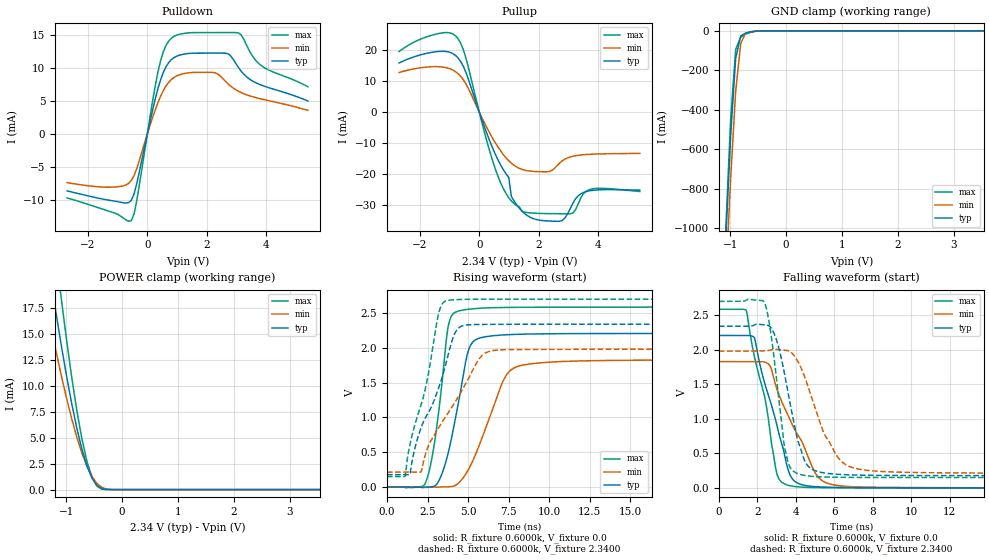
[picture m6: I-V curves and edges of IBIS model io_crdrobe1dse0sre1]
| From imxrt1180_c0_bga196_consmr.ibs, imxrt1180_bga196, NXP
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[Model]  io_crdrobe1dse0sre1
|   Model io_crdrobe1dse0sre1
| This model was characterised for following simulation conditions:
| External (pad) voltage:
|   - Typ: 2.34V,   - Min: 1.98V,   - Max: 2.7V
| Library cells for typ/min/max conditions are connected as defined below:
|  PAD_IO - External Pad
|  ipp_do - Core Input
|  ipp_obe - Output Buffer Enable
|  ASRCN3V3[3] - NC
|  ASRCN3V3[4] - NC
|  ASRCP3V3[4] - NC
|  REFAPBIAS3V3 - gnde
|  REFBAMPL3V3 - vdd1v8
|  REFCAMPH3V3 - vdd1v8
|  REFDNBIAS3V3 - vdd1v8
|  REFH3V3 - REFH3V3
|  REFL3V3 - REFL3V3
|  gnde - gnde
|  ipp_dse - gnde
|  ipp_ina235_3v - NC
|  ipp_ina40_3v - NC
|  ipp_ina_mux - NC
|  ipp_ind - NC
|  ipp_ind_1p8v - NC
|  ipp_ind_3v - NC
|  ipp_sre - vdd
|  vdd - vdd
|  vdd1v8 - vdd1v8
|  vdda - vdde3v3
|  vdde3v3 - vdde3v3
| All other pins connected to ground
Model_type I/O
Polarity   Non-Inverting
Enable   Active-High
Vinl =   0.7020V
Vinh =   1.6300V
Vmeas =  1.1700V
Cref =   15.0000pF
Rref =   0.6000k
Vref =   0.0V
C_comp   3.9951pF   3.8194pF   4.1033pF
|C_comp_pullup   0.5141pF   0.5881pF   0.4995pF
|C_comp_pulldown   2.0717pF   2.1609pF   1.8543pF
[Model Spec]
| variable   typ   min   max
Vinh   1.6300V   NA   NA
Vinl   0.7020V   NA   NA
Vref   0.0V   0.0V   0.0V
Cref   15.0000pF   15.0000pF   15.0000pF
Rref   0.6000k   0.6000k   0.6000k
[Receiver Thresholds]
Vcross_high  =   0.0V
Vcross_low  =   0.0V
Vdiff_ac  =   0.0V
Vdiff_dc  =   0.0V
Tdiffslew_ac  =   0.0S
[Temperature Range]   25.0000   0.1250k   -40.0000
[Voltage Range]   2.3400V   1.9800V   2.7000V
[Pullup Reference]   2.3400V   1.9800V   2.7000V
[Pulldown Reference]   0.0V   0.0V   0.0V
[POWER Clamp Reference]   2.3400V   1.9800V   2.7000V
[GND Clamp Reference]   0.0V   0.0V   0.0V
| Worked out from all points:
|   slope of the pulldown table from 0 to 0.351 V, typ, clamps not added: 51.9 ohm
|   slope of the pullup table from 0 to 0.351 V, typ, clamps not added: 37.8 ohm
|   GND clamp passes 1 mA (typ) near -0.49 V on its own axis
|   POWER clamp passes 1 mA (typ) near -0.53 V on its own axis
|   rising waveform, R_fixture 0.6000k, V_fixture 0.0: 20-80 % time 1.1ns typ, 1.77ns min, 787ps max; typ from 0 V to 2.21 V
|   rising waveform, R_fixture 0.6000k, V_fixture 2.3400: 20-80 % time 2ns typ, 2.66ns min, 1.49ns max; typ from 0.177 V to 2.34 V
|   falling waveform, R_fixture 0.6000k, V_fixture 0.0: 20-80 % time 1.29ns typ, 1.78ns min, 1.09ns max; typ from 2.21 V to 0 V
|   falling waveform, R_fixture 0.6000k, V_fixture 2.3400: 20-80 % time 975ps typ, 1.48ns min, 648ps max; typ from 2.34 V to 0.177 V
[Pulldown]
|Voltage   I(typ)   I(min)   I(max)
-2.7V     -8.67mA    -7.41mA    -9.74mA
-1.17V    -10.17mA   -8.095mA   -11.93mA
-540mV    -10.08mA   -7.082mA   -13.18mA
-360mV    -7.618mA   -5.325mA   -10.21mA
360mV     6.913mA    4.777mA    9.448mA
630mV     10.2mA     7.277mA    13.44mA
900mV     11.57mA    8.553mA    14.79mA
2.25V     12.24mA    9.288mA    15.36mA
2.7V      12.17mA    7.637mA    15.36mA
3.06V     10.09mA    6.461mA    15.32mA
3.78V     7.479mA    5.34mA     10.54mA
5.4V      4.985mA    3.556mA    7.138mA
[Pullup]
|Voltage   I(typ)   I(min)   I(max)
-2.7V     15.88mA    12.82mA    19.56mA
-1.44V    19.54mA    14.7mA     25.24mA
-720mV    17.58mA    12.48mA    23.82mA
-450mV    12.84mA    9.141mA    17.52mA
630mV     -15.42mA   -11.25mA   -20.73mA
990mV     -21.04mA   -15.7mA    -27.62mA
1.08V     -27.24mA   -16.49mA   -28.69mA
1.44V     -31.99mA   -18.49mA   -32.03mA
2.7V      -35.24mA   -16.46mA   -32.81mA
3.15V     -29.4mA    -14.24mA   -32.57mA
3.51V     -25.93mA   -13.74mA   -26.26mA
5.4V      -25.18mA   -13.3mA    -25.63mA
[GND_clamp]
|Voltage   I(typ)   I(min)   I(max)
-2.7V     -12.91A    -12.88A    -13.56A
-1.08V    -1.077A    -1.286A    -1.025A
-990mV    -533.6mA   -749.4mA   -449.1mA
-900mV    -139.2mA   -307mA     -94.25mA
-810mV    -25.49mA   -63.91mA   -32.87mA
-720mV    -11.78mA   -11.41mA   -16.65mA
-540mV    -1.684mA   -1.901mA   -2.149mA
-360mV    -36.04uA   -133.3uA   -15.05uA
5.4V      0A         0A         0A
[POWER_clamp]
|Voltage   I(typ)   I(min)   I(max)
-2.7V     73.96mA    57.58mA    95.4mA
-1.44V    26.15mA    20.18mA    34.67mA
-1.35V    22.86mA    17.7mA     30.34mA
-1.26V    19.66mA    15.3mA     26.09mA
-1.17V    16.56mA    12.98mA    21.97mA
-1.08V    13.59mA    10.78mA    17.99mA
-900mV    8.212mA    6.776mA    10.73mA
-720mV    3.9mA      3.518mA    4.888mA
-630mV    2.284mA    2.252mA    2.724mA
-540mV    1.103mA    1.268mA    1.195mA
-360mV    77.93uA    204.3uA    41.52uA
5.4V      0A         0A         0A
[Ramp]
| variable   typ   min   max
dV/dt_r  1.3244/1.0982n   1.0970/1.7718n   1.5519/0.7865n
dV/dt_f  1.2978/0.9748n   1.0605/1.4843n   1.5299/0.6476n
R_load = 0.6000k
[Rising Waveform]
R_fixture= 0.6000k
V_fixture= 0.0
V_fixture_min= 0.0
V_fixture_max= 0.0
|time   V(typ)   V(min)   V(max)
0s        133.2nV    3.451uV    44.06nV
2.399ns   -1.746mV   -5.701mV   74.77mV
2.994ns   21.55mV    -2.011mV   736mV
3.785ns   499.2mV    2.221mV    2.32V
4.667ns   1.562V     123.1mV    2.543V
5.021ns   1.966V     250.8mV    2.554V
5.443ns   2.114V     457.5mV    2.564V
7.306ns   2.187V     1.588V     2.58V
8.814ns   2.199V     1.769V     2.583V
60ns      2.207V     1.828V     2.587V
[Rising Waveform]
R_fixture= 0.6000k
V_fixture= 2.3400
V_fixture_min= 1.9800
V_fixture_max= 2.7000
|time   V(typ)   V(min)   V(max)
0s        177mV      212.5mV    150.2mV
1.117ns   176mV      212.4mV    151.9mV
1.418ns   183.8mV    211.9mV    614.9mV
2.104ns   853.1mV    216.7mV    1.183V
3.169ns   1.414V     847.7mV    2.479V
3.727ns   1.859V     1.049V     2.682V
4.48ns    2.299V     1.331V     2.695V
5.79ns    2.336V     1.874V     2.699V
6.922ns   2.338V     1.97V      2.7V
60ns      2.34V      1.98V      2.7V
[Falling Waveform]
R_fixture= 0.6000k
V_fixture= 0.0
V_fixture_min= 0.0
V_fixture_max= 0.0
|time   V(typ)   V(min)   V(max)
0s        2.207V     1.828V     2.586V
1.408ns   2.208V     1.828V     2.572V
1.833ns   2.176V     1.827V     1.919V
2.393ns   1.502V     1.819V     1.296V
2.634ns   1.291V     1.774V     858.9mV
3.031ns   887.7mV    1.415V     188.5mV
3.887ns   108.2mV    871.6mV    21.14mV
5.174ns   14.22mV    150.9mV    3.217mV
6.696ns   4.267mV    19.97mV    526.3uV
60ns      6.17uV     16.82uV    1.377uV
[Falling Waveform]
R_fixture= 0.6000k
V_fixture= 2.3400
V_fixture_min= 1.9800
V_fixture_max= 2.7000
|time   V(typ)   V(min)   V(max)
0s        2.34V      1.98V      2.7V
2.373ns   2.359V     1.985V     2.679V
2.954ns   2.175V     2.006V     1.677V
3.375ns   1.702V     1.995V     652.7mV
3.559ns   1.43V      1.989V     405.2mV
4.06ns    728.7mV    1.852V     210.3mV
4.544ns   348.3mV    1.539V     175.9mV
6.132ns   196.6mV    462mV      153.3mV
7.882ns   181.8mV    248.3mV    150.6mV
60ns      177mV      212.6mV    150.2mV
